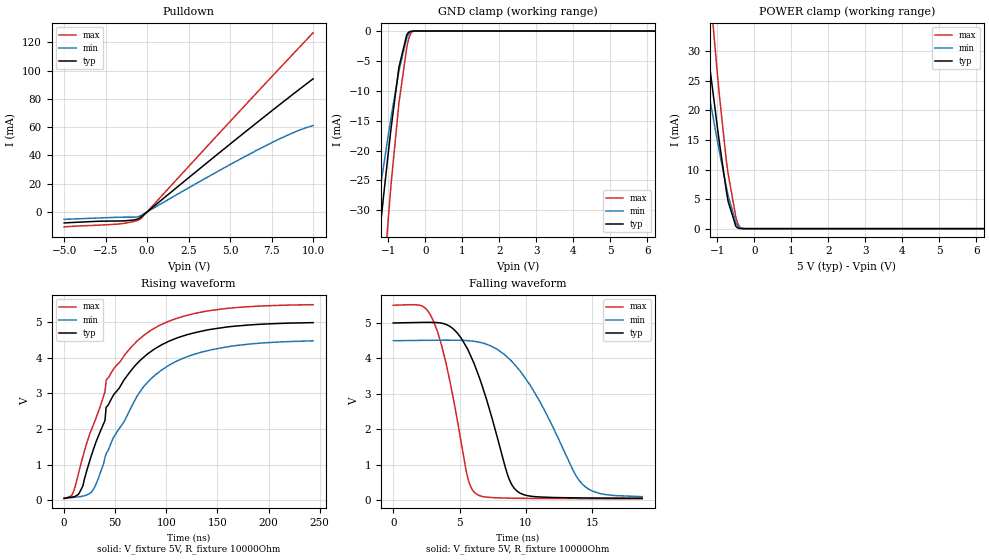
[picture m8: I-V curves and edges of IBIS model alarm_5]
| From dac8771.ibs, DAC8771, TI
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|   alarm_5 Model
[Model]   alarm_5
Model_type   Open_drain
Polarity   Inverting
Vmeas = 2.5
Vref = 5
Cref = 2pF
Rref = 10000
|   typ   min   max
|   (nom PVT)   (fast PVT)   (slow PVT)
C_comp   2.259e-12   2.193e-12   2.401e-12
| Where nom  PVT is Nominal Process, 5V, 27C
|   Fast PVT is Strong Process,  5.5V, -40C
|   Slow PVT is Weak Process,   4.5V, 150C
[Voltage Range]   5   4.5   5.5
|Junction Temperature
[Temperature Range]   27   150   -40
[Pullup Reference]   5   4.5   5.5
[Pulldown Reference]   0   0   0
[Power Clamp Reference]   5   4.5   5.5
[GND Clamp Reference]   0   0   0
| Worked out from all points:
|   slope of the pulldown table from 0 to 0.75 V, typ, clamps not added: 103 ohm
|   GND clamp passes 1 mA (typ) near -0.51 V on its own axis
|   POWER clamp passes 1 mA (typ) near -0.53 V on its own axis
|   falling waveform, V_fixture 5V, R_fixture 10000Ohm: 20-80 % time 2.45ns typ, 3.77ns min, 1.74ns max; typ from 5 V to 0.061 V
|   rising waveform, V_fixture 5V, R_fixture 10000Ohm: 20-80 % time 52.9ns typ, 54.9ns min, 51.6ns max; typ from 0.051 V to 4.98 V
[Pulldown]
|   Voltage   I(typ)   I(min)   I(max)
-5V       -7.781mA   -5.248mA   -10.56mA
-1.65V    -6.406mA   -3.757mA   -8.468mA
-806mV    -5.703mA   -3.692mA   -6.782mA
-396.5mV  -3.789mA   -2.683mA   -4.877mA
3.172V    30.66mA    21.56mA    40.8mA
6.317V    60.49mA    41.87mA    80.78mA
8.779V    83.27mA    56.03mA    111.7mA
10V       94.25mA    61.15mA    126.8mA
[GND Clamp]
|   Voltage   I(typ)   I(min)   I(max)
-5V       -1.657A    -1.239A    -1.964A
-1.845V   -71.48mA   -53.72mA   -103mA
-1.175V   -30.54mA   -24.7mA    -45.66mA
-1.005V   -20.8mA    -17.74mA   -32.02mA
-919mV    -16.11mA   -14.34mA   -25.44mA
-710mV    -6.06mA    -6.671mA   -12.07mA
-500mV    -666uA     -1.167mA   -2.833mA
-451.5mV  -245.9uA   -552uA     -1.46mA
-405.5mV  -76.18uA   -225.2uA   -598.2uA
-352.5mV  -16.31uA   -67.06uA   -139.6uA
-266mV    -931.7nA   -7.61uA    -5.754uA
10V       0A         0A         0A
[POWER Clamp]
|   Voltage   I(typ)   I(min)   I(max)
-5V       1.619A     1.21A      1.916A
-2.15V    77.85mA    57.36mA    112.9mA
-1.184V   26.43mA    21.35mA    39.46mA
-990mV    16.81mA    14.61mA    25.7mA
-950mV    14.91mA    13.26mA    22.99mA
-754mV    6.348mA    7.009mA    11.43mA
-705mV    4.58mA     5.584mA    9.251mA
-500mV    438.7uA    1.082mA    2.063mA
-429.5mV  87.44uA    385.8uA    671.6uA
-358mV    11.34uA    103.2uA    101.9uA
-239mV    207.1nA    7.214uA    1.07uA
10V       0A         0A         0A
[Ramp]
R_load = 10000
|   typ   min   max
dV/dt_r   2.96933/4.91744e-08   2.66114/5.15742e-08   3.27454/4.78046e-08
dV/dt_f   2.96943/2.45736e-09   2.66135/3.79038e-09   3.2746/1.74028e-09
[Falling Waveform]
V_fixture = 5V
V_fixture_min = 4.5V
V_fixture_max = 5.5V
R_fixture = 10000Ohm
|   Time   V(typ)   V(min)   V(max)
0s        5V         4.5V       5.5V
2.202ns   5.016V     4.51V      5.475V
3.049ns   5.014V     4.513V     5.044V
3.97ns    4.961V     4.515V     3.887V
5.617ns   4.259V     4.502V     641.8mV
6.18ns    3.778V     4.479V     204.5mV
8.628ns   718.6mV    4.028V     62.91mV
9.394ns   244.5mV    3.725V     58.07mV
14.3ns    68.15mV    446.8mV    48.56mV
18.78ns   60.57mV    103.5mV    46.71mV
[Rising Waveform]
V_fixture = 5V
V_fixture_min = 4.5V
V_fixture_max = 5.5V
R_fixture = 10000Ohm
|   Time   V(typ)   V(min)   V(max)
0s        50.94mV    64.35mV    42.32mV
8.547ns   90.58mV    75.96mV    203.5mV
18.43ns   409mV      115.1mV    1.233V
29.79ns   1.52V      360.3mV    2.197V
40ns      2.239V     1.201V     3.044V
41.18ns   2.607V     1.309V     3.374V
78.02ns   4.014V     3.188V     4.626V
101.6ns   4.445V     3.768V     5.009V
133.8ns   4.736V     4.148V     5.272V
243.7ns   4.98V      4.47V      5.484V
